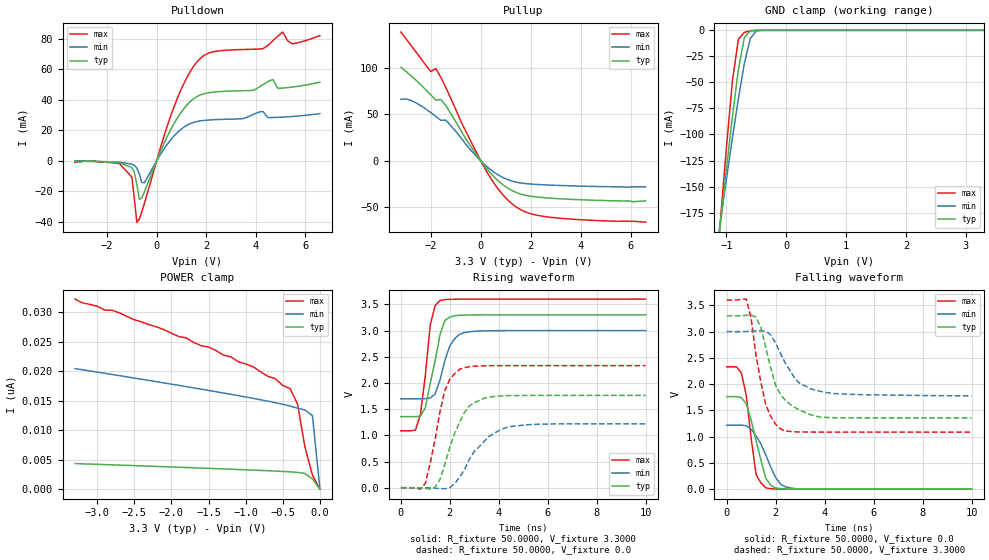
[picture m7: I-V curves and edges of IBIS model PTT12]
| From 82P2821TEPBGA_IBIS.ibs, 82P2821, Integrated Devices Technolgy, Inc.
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|   Model PTT12
[Model]		PTT12
Model_type	3-state
Polarity   Non-Inverting
Enable   Active-Low
C_comp   6.2400pF   5.8600pF   7.2200pF
[Temperature Range]	  25.0000   90.0000   -40.0000
[Voltage Range]   3.3000V   3.0000V   3.6000V
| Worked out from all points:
|   slope of the pulldown table from 0 to 0.495 V, typ, clamps not added: 27.3 ohm
|   slope of the pullup table from 0 to 0.495 V, typ, clamps not added: 30.5 ohm
|   GND clamp passes 1 mA (typ) near -0.61 V on its own axis
|   rising waveform, R_fixture 50.0000, V_fixture 3.3000: 20-80 % time 501ps typ, 522ps min, 348ps max; typ from 1.36 V to 3.3 V
|   rising waveform, R_fixture 50.0000, V_fixture 0.0: 20-80 % time 839ps typ, 1.13ns min, 606ps max; typ from 0 V to 1.76 V
|   falling waveform, R_fixture 50.0000, V_fixture 0.0: 20-80 % time 578ps typ, 729ps min, 383ps max; typ from 1.76 V to 0 V
|   falling waveform, R_fixture 50.0000, V_fixture 3.3000: 20-80 % time 815ps typ, 940ps min, 570ps max; typ from 3.3 V to 1.36 V
[Pulldown]
|Voltage	  I(typ)   I(min)   I(max)
-3.3V     0A         0A         -1mA
-1.5V     -1.3mA     -900uA     -1.9mA
-1V       -4.4mA     -2.2mA     -10.7mA
-800mV    -15.42mA   -4.67mA    -40.26mA
-700mV    -25.31mA   -8.49mA    -38.22mA
-600mV    -24.49mA   -14.21mA   -33.52mA
700mV     24.37mA    16.23mA    35.28mA
1.7V      42.75mA    26.06mA    66.19mA
4.3V      50.03mA    32.37mA    73.58mA
5.1V      47.79mA    28.72mA    84.5mA
5.5V      48.45mA    29.12mA    76.76mA
6.6V      51.62mA    30.97mA    82.16mA
[Pullup]
|Voltage	  I(typ)   I(min)   I(max)
-3.2V     100.7mA    66.22mA    138.6mA
-2.8V     91.81mA    65.09mA    124.6mA
-2V       70.88mA    51.92mA    96.06mA
-1.8V     65.41mA    47.77mA    99.32mA
-1.6V     66.07mA    43.67mA    89.98mA
-1.4V     59.58mA    43.76mA    78.99mA
-700mV    28.09mA    21.46mA    37.07mA
200mV     -7.125mA   -5.115mA   -9.891mA
700mV     -21.57mA   -15.14mA   -30.44mA
1.3V      -32.63mA   -22.12mA   -47.27mA
2.6V      -39.77mA   -25.86mA   -60.06mA
6.6V      -43mA      -28mA      -66mA
[GND_clamp]
|Voltage	  I(typ)   I(min)   I(max)
-3.3V     -1.417A    -1.129A    -1.858A
-1.2V     -239.1mA   -224.9mA   -255mA
-1.1V     -185.6mA   -183.6mA   -182.5mA
-1V       -133.2mA   -143mA     -112.6mA
-900mV    -82.99mA   -103.4mA   -48.97mA
-800mV    -37.69mA   -65.64mA   -8.507mA
-700mV    -7.019mA   -31.73mA   -1.941mA
-600mV    -418.3uA   -7.667mA   -417.7uA
-500mV    -26.63uA   -550.4uA   -45.83uA
3.3V      768.1fA    13.73nA    -711.9pA
[POWER_clamp]
|Voltage	  I(typ)   I(min)   I(max)
-3.3V     4.336nA    20.42nA    32.21nA
-2.9V     4.166nA    19.63nA    30.35nA
-2.7V     4.073nA    19.23nA    29.87nA
-1.6V     3.575nA    16.95nA    24.31nA
-1.5V     3.528nA    16.73nA    24.07nA
-1.1V     3.334nA    15.85nA    21.6nA
-900mV    3.232nA    15.39nA    20.75nA
-400mV    2.936nA    14.08nA    17.03nA
-300mV    2.841nA    13.73nA    14.41nA
-200mV    2.659nA    13.4nA     7.085nA
-100mV    1.727nA    12.47nA    2.401nA
0V        774.4fA    199.7pA    530.4fA
[Ramp]
| variable   typ   min   max
dV/dt_r		1.0566/0.8255n   0.7314/1.1207n   1.3980/0.5545n
dV/dt_f		1.1658/0.8000n   0.7344/0.9742n   1.5084/0.5079n
R_load =	50.0000
[Rising Waveform]
R_fixture=	50.0000
V_fixture=	3.3000
V_fixture_min=	3.0000
V_fixture_max=	3.6000
|time   V(typ)   V(min)   V(max)
0s        1.357V     1.697V     1.086V
600ps     1.357V     1.697V     1.101V
800ps     1.362V     1.697V     1.399V
1ns       1.526V     1.698V     2.146V
1.2ns     1.99V      1.711V     3.104V
1.4ns     2.425V     1.79V      3.475V
1.6ns     2.922V     2.058V     3.571V
2ns       3.254V     2.705V     3.595V
2.6ns     3.293V     2.962V     3.599V
10ns      3.299V     2.999V     3.599V
[Rising Waveform]
R_fixture=	50.0000
V_fixture=	0.0
V_fixture_min=	0.0
V_fixture_max=	0.0
|time   V(typ)   V(min)   V(max)
0s        0V         0V         0V
800ps     -2.657mV   83.09uV    -27.84mV
1ns       -14.36mV   -643.4uV   81.4mV
1.4ns     9.12mV     -8.851mV   929.3mV
1.8ns     453mV      -19.32mV   1.861V
2.4ns     1.25V      198.6mV    2.261V
3ns       1.622V     692.8mV    2.318V
3.6ns     1.724V     979.1mV    2.328V
4.4ns     1.757V     1.161V     2.33V
10ns      1.761V     1.219V     2.33V
[Falling Waveform]
R_fixture=	50.0000
V_fixture=	0.0
V_fixture_min=	0.0
V_fixture_max=	0.0
|time   V(typ)   V(min)   V(max)
0s        1.761V     1.219V     2.33V
400ps     1.762V     1.22V      2.329V
600ps     1.742V     1.22V      2.212V
800ps     1.625V     1.208V     1.785V
1.2ns     921.7mV    1.014V     279.5mV
1.6ns     206.2mV    650.3mV    24.39mV
1.8ns     73.11mV    417.8mV    9.461mV
2.2ns     11.08mV    95.41mV    1.126mV
2.8ns     858uV      9.209mV    110.8uV
10ns      7.143uV    6.826uV    1.834uV
[Falling Waveform]
R_fixture=	50.0000
V_fixture=	3.3000
V_fixture_min=	3.0000
V_fixture_max=	3.6000
|time   V(typ)   V(min)   V(max)
0s        3.3V       3V         3.6V
800ps     3.31V      3.001V     3.619V
1ns       3.315V     3.005V     3.242V
1.2ns     3.275V     3.013V     2.542V
1.6ns     2.687V     3.009V     1.601V
2ns       1.975V     2.778V     1.236V
2.2ns     1.8V       2.583V     1.146V
3ns       1.502V     2.004V     1.089V
3.8ns     1.374V     1.865V     1.087V
10ns      1.357V     1.776V     1.086V
